(* Logix 5000 AddOnInstructionDefinition export Banner_Q76_PD_v4; software revision 33.00 *)

TYPE Banner_Q76_PDIO_v4 :   // UDT with all of the variables needed to control an IO-Link Q76 version.
STRUCT
   Set0 : Banner_Q76_Set0_v4;
   Set1 : Banner_Q76_Set1_v4;
   PDO : SINT;
END_STRUCT
END_TYPE

TYPE Banner_Q76_Set0_v4 :
STRUCT
   Q : SINT;
   Warning : SINT;
   Status : SINT;
END_STRUCT
END_TYPE

TYPE Banner_Q76_Set1_v4 :
STRUCT
   Q : SINT;
   Signal : INT;
END_STRUCT
END_TYPE

ADD_ON_INSTRUCTION Banner_Q76_PD_v4   (* revision 4.0, vendor Banner Engineering *)
// AOI used for Q76.
VAR_IN_OUT
   Process_Data : Banner_Q76_PDIO_v4; {required}
END_VAR
VAR_INPUT
   PDI_Byte : SINT; {required}
END_VAR
VAR_IN_OUT
   PDO_Byte : SINT; {required}
END_VAR
VAR_INPUT
   PDI_Content : SINT; {required}
END_VAR
VAR
   Temp : INT[3]; {access None}
END_VAR

ROUTINE Logic   (* ladder *)
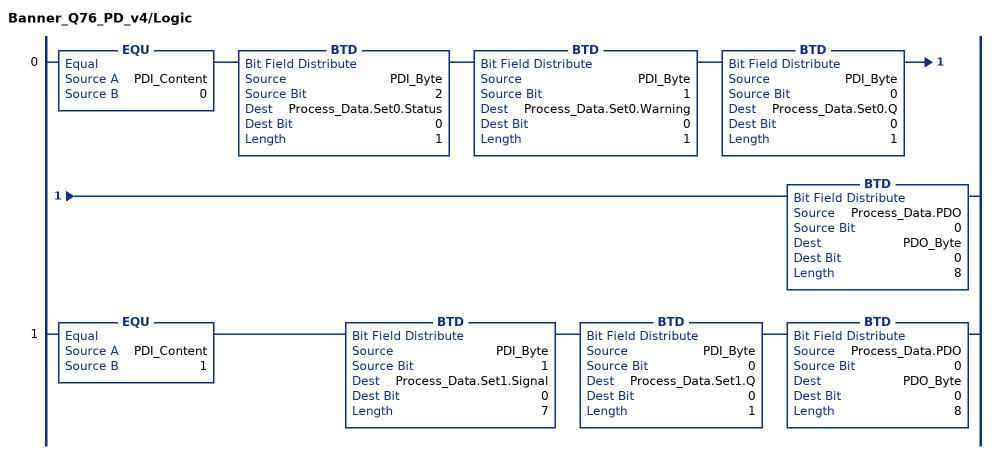
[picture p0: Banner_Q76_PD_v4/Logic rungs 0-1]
   0: EQU(PDI_Content,0)BTD(PDI_Byte,2,Process_Data.Set0.Status,0,1)BTD(PDI_Byte,1,Process_Data.Set0.Warning,0,1)BTD(PDI_Byte,0,Process_Data.Set0.Q,0,1)BTD(Process_Data.PDO,0,PDO_Byte,0,8);
   1: EQU(PDI_Content,1)BTD(PDI_Byte,1,Process_Data.Set1.Signal,0,7)BTD(PDI_Byte,0,Process_Data.Set1.Q,0,1)BTD(Process_Data.PDO,0,PDO_Byte,0,8);
END_ROUTINE
END_ADD_ON_INSTRUCTION
